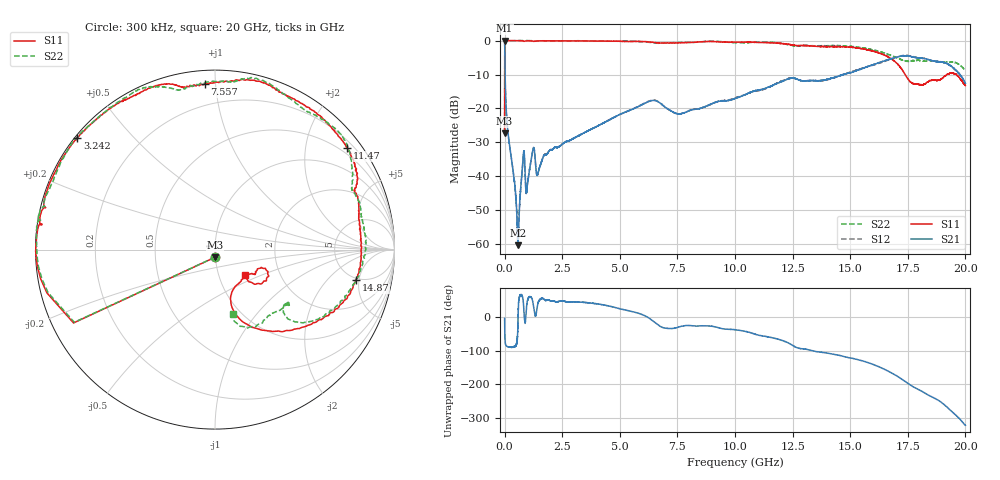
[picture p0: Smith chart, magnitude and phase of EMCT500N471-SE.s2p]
!EMCT500N471
!Johanson Technology Inc.
!www.johansontechnology.com
!Test Board Conditions:
!Substrate Type  RO4350B
!Substrate Thickness  10 mil
!Substrate Dk  3.66
!TL Type: GCPW
!TL Trace Width  22 mil
!TL Gap  14 mil
!PART MODE SINGLE ENDED (AKA BYPASS)
!DUT TOPOLOGY	SERIES-SHUNT
# MHz S  dB  R 50
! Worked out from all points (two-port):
!   20001 points, 300 kHz to 20 GHz, reference 50 ohm
!   highest |S21| = -0.02 dB at 300 kHz (marker M1); lowest = -60.3 dB at 575.3 MHz (marker M2)
!   |S21| within 3 dB of the highest: start of sweep to 6.902 MHz
!   lowest |S11| = -27.3 dB at 300 kHz (marker M3), VSWR 1.09, Z = 49.8 - j4.28 ohm
!   |S11| at or under -10 dB: start of sweep to 2.307 MHz; 17.38 GHz to 19.2 GHz (1.812 GHz wide, 9.9 % of centre); 19.6 GHz to end of sweep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
!   |S22| runs from -27.4 to 0.0 dB; largest |S21 - S12| = 0.015
!   S11 on the Smith chart (normalised r, x): 300 kHz: 1.00, -0.09; 3.242 GHz: 0.01, +0.36; 7.557 GHz: 0.07, +0.94; 11.47 GHz: 0.35, +2.90; 14.87 GHz: 4.71, -4.55; 20 GHz: 1.34, -0.39
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0.3  -27.34 -90.7  -0.02 -2.6  -0.01 -2.5  -27.39 -90.8
105.298  -0.03 -177.4  -23.98 -86.7  -23.94 -86.8  -0.08 -177.3
575.291  -0.04 174.9  -60.31 -24.1  -59.02 -24.9  -0.00 174.1
644.29  -0.05 174.0  -49.30 62.8  -49.28 60.7  0.01 173.2
787.288  -0.09 172.0  -36.05 58.8  -36.13 58.6  -0.02 170.9
992.285  -0.09 170.2  -42.20 50.8  -42.22 50.5  -0.00 168.9
1224.282  -0.16 166.3  -32.29 47.3  -32.30 47.6  -0.10 166.1
1454.278  -0.10 164.5  -38.94 44.0  -38.87 43.9  -0.09 164.1
1946.271  -0.06 157.5  -32.39 51.6  -32.33 51.6  -0.17 157.9
3242.251  -0.10 140.9  -27.90 46.2  -27.93 46.1  -0.06 142.5
3334.25  -0.12 139.9  -27.59 45.9  -27.57 46.0  -0.05 141.5
6667.2  -0.70 101.5  -18.03 -22.6  -17.99 -23.0  -0.80 102.8
7557.187  -0.67 93.5  -21.62 -28.6  -21.62 -28.5  -0.57 91.1
10000.15  -0.48 61.5  -17.09 -36.7  -16.89 -36.8  -0.62 60.1
11472.13  -0.65 37.6  -13.63 -58.7  -13.73 -57.7  -0.48 40.8
13334.1  -1.63 15.0  -11.80 -99.3  -11.79 -99.5  -1.51 14.3
14870.08  -1.89 -12.3  -9.69 -119.1  -9.61 -118.0  -1.66 -4.9
16667.05  -4.91 -53.3  -5.58 -161.5  -5.66 -160.3  -4.12 -40.7
17398.04  -10.15 -73.4  -4.50 167.5  -4.39 167.8  -6.03 -40.7
18430.02  -11.85 -32.6  -5.71 126.2  -5.70 125.8  -6.07 -38.6
19219.01  -9.91 -22.5  -6.83 90.5  -6.90 90.1  -6.38 -53.0
20000  -13.26 -39.8  -12.59 36.6  -12.72 37.2  -8.68 -73.9
